FUNCTION "FC_VALVE_MT" : VOID
TITLE =VALVE
{ S7_language := '9(1) Angielski (Stany Zjednoczone)  11.01.2022  09:45:15' }
VERSION : 0.1


VAR_INPUT
  REL_CONTROL : BOOL ;	//RELEASE FOR CONTROLL
  RES_ALARM : BOOL ;	//RESET ALARMS
  PBS : BOOL ;	//PROTECTION VALVE
  Pos_Valve : REAL ;
END_VAR
VAR_IN_OUT
  DDB : "UDT_VALVE_MT";
END_VAR
BEGIN
NETWORK
TITLE =ANALOG VALVE



NETWORK
TITLE =MANUAL MODE / AUTOMATIC MODE
//MANUAL MODE
      U(    ;
      U(    ;
      O     #DDB.CW.Open;
      O     #DDB.CW.Close;
      )     ;
      S     #DDB.SM.ManualMode;
      U(    ;
      O     #REL_CONTROL;
      ON    #REL_CONTROL;
      )     ;
      U     #DDB.CW.AStart;
      FP    #DDB.SM.SM_Shot1;
      R     #DDB.SM.ManualMode;
      U     #DDB.SM.ManualMode;
      )     ;
      NOT   ;
      =     #DDB.SM.AutomaticMode;
NETWORK
TITLE =
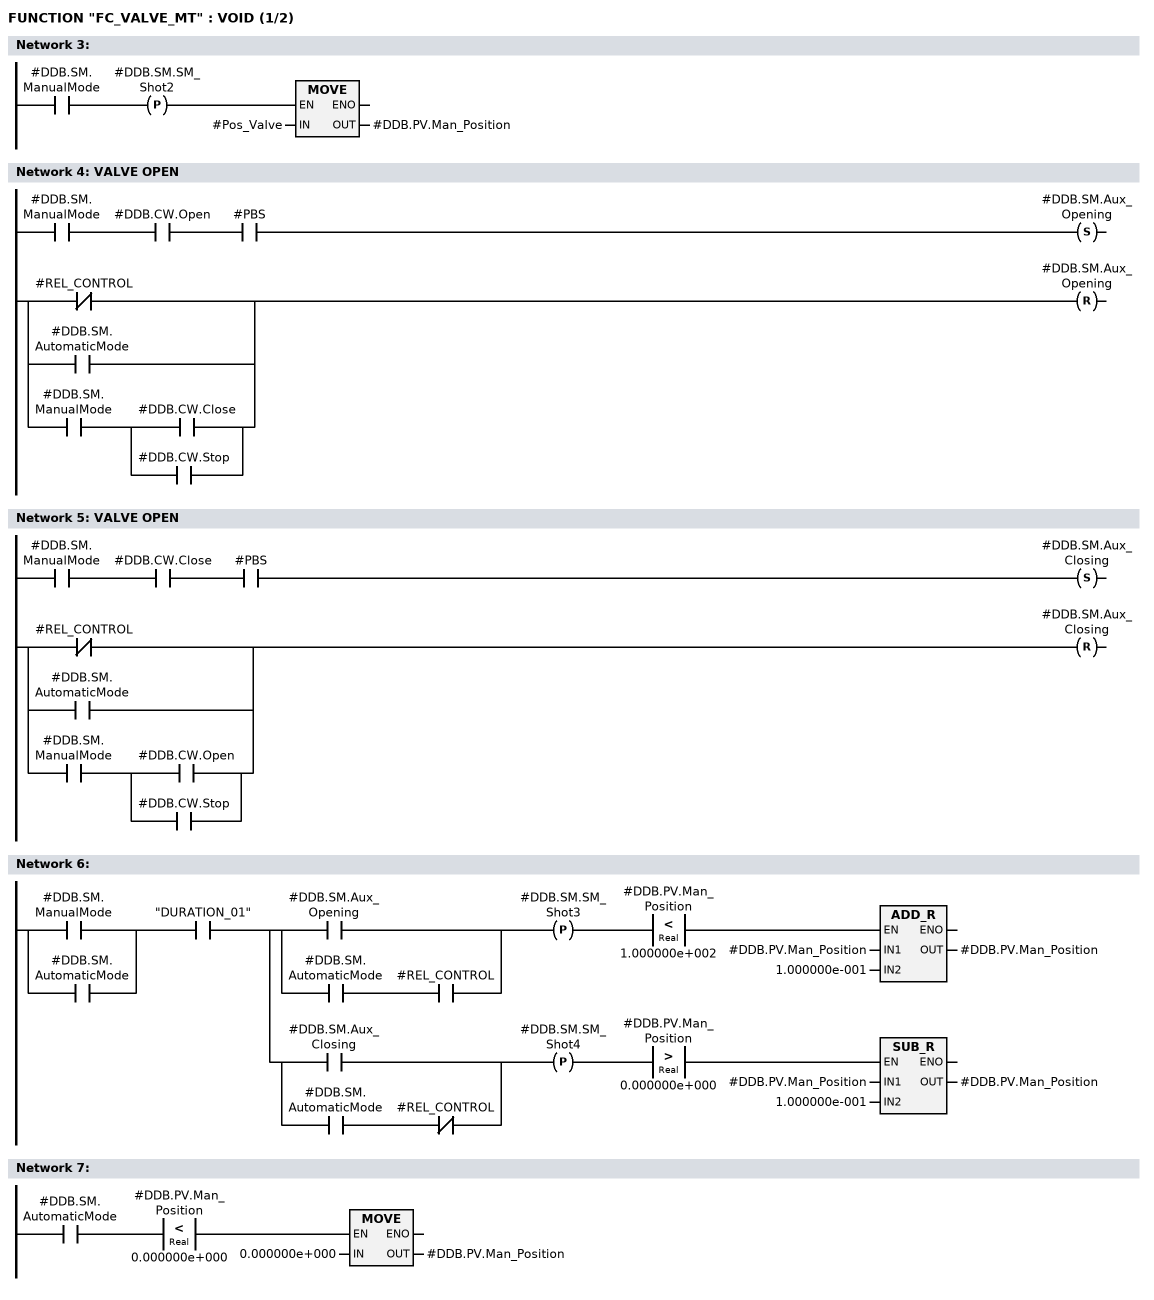
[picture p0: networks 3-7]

      U     #DDB.SM.ManualMode;
      FP    #DDB.SM.SM_Shot2;
      SPBNB _001;
      L     #Pos_Valve;
      T     #DDB.PV.Man_Position;
_001: NOP   0;
NETWORK
TITLE =VALVE OPEN

      U     #DDB.SM.ManualMode;
      U     #DDB.CW.Open;
      U     #PBS;
      S     #DDB.SM.Aux_Opening;
      U(    ;
      ON    #REL_CONTROL;
      O     #DDB.SM.AutomaticMode;
      O     ;
      U     #DDB.SM.ManualMode;
      U(    ;
      O     #DDB.CW.Close;
      O     #DDB.CW.Stop;
      )     ;
      )     ;
      R     #DDB.SM.Aux_Opening;
      NOP   0;
NETWORK
TITLE =VALVE OPEN

      U     #DDB.SM.ManualMode;
      U     #DDB.CW.Close;
      U     #PBS;
      S     #DDB.SM.Aux_Closing;
      U(    ;
      ON    #REL_CONTROL;
      O     #DDB.SM.AutomaticMode;
      O     ;
      U     #DDB.SM.ManualMode;
      U(    ;
      O     #DDB.CW.Open;
      O     #DDB.CW.Stop;
      )     ;
      )     ;
      R     #DDB.SM.Aux_Closing;
      NOP   0;
NETWORK
TITLE =


      U(    ;
      O     #DDB.SM.ManualMode;
      O     #DDB.SM.AutomaticMode;
      )     ;
      U     "DURATION_01";
      =     L      0.0;
      U     L      0.0;
      U(    ;
      O     #DDB.SM.Aux_Opening;
      O     ;
      U     #DDB.SM.AutomaticMode;
      U     #REL_CONTROL;
      )     ;
      FP    #DDB.SM.SM_Shot3;
      U(    ;
      L     #DDB.PV.Man_Position;
      L     1.000000e+002;
      <R    ;
      )     ;
      SPBNB _002;
      L     #DDB.PV.Man_Position;
      L     1.000000e-001;
      +R    ;
      T     #DDB.PV.Man_Position;
_002: NOP   0;
      U     L      0.0;
      U(    ;
      O     #DDB.SM.Aux_Closing;
      O     ;
      U     #DDB.SM.AutomaticMode;
      UN    #REL_CONTROL;
      )     ;
      FP    #DDB.SM.SM_Shot4;
      U(    ;
      L     #DDB.PV.Man_Position;
      L     0.000000e+000;
      >R    ;
      )     ;
      SPBNB _003;
      L     #DDB.PV.Man_Position;
      L     1.000000e-001;
      -R    ;
      T     #DDB.PV.Man_Position;
_003: NOP   0;
NETWORK
TITLE =

      U     #DDB.SM.AutomaticMode;
      U(    ;
      L     #DDB.PV.Man_Position;
      L     0.000000e+000;
      <R    ;
      )     ;
      SPBNB _004;
      L     0.000000e+000;
      T     #DDB.PV.Man_Position;
_004: NOP   0;
NETWORK
TITLE =

NETWORK
TITLE =
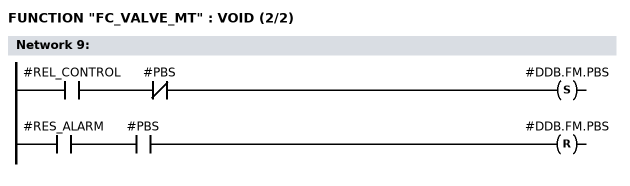
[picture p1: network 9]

      U     #REL_CONTROL;
      UN    #PBS;
      S     #DDB.FM.PBS;
      U     #RES_ALARM;
      U     #PBS;
      R     #DDB.FM.PBS;
      NOP   0;
NETWORK
TITLE =

NETWORK
TITLE =VISU STATUS


      U     #DDB.FM.PBS;
      =     #DDB.SM.GeneralError;
      CLR   ;
      =     #DDB.SM.GeneralWarning;

      U     #REL_CONTROL;
      =     #DDB.SM.Release;

END_FUNCTION

